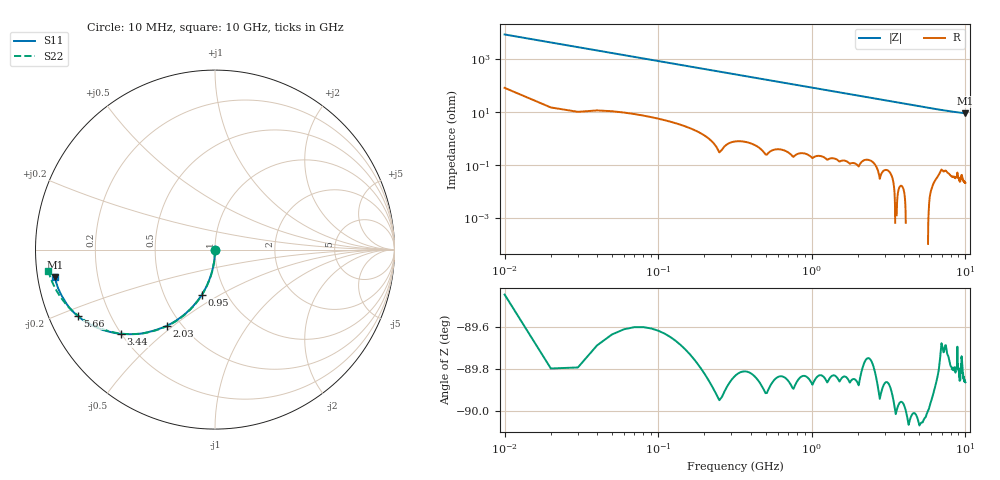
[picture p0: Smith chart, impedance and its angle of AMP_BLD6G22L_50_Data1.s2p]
! Created Fri Sep 09 16:33:03 2011
# ghz S ma R 50
! 2 Port Network Data from SP1.SP block
! freq  magS11  angS11  magS21  angS21  magS12  angS12  magS22  angS22
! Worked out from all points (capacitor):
!   1000 points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, 10 MHz to 10 GHz, reference 50 ohm
!   read as one part in shunt: C = 1.87 pF near 60 MHz
!   lowest |Z| = 9.03 ohm at 10 GHz (marker M1)
!   S11 on the Smith chart (normalised r, x): 10 MHz: 1.00, -0.01; 950 MHz: 0.77, -0.41; 2.03 GHz: 0.42, -0.47; 3.44 GHz: 0.20, -0.37; 5.66 GHz: 0.09, -0.23; 10 GHz: 0.05, -0.08
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0.01  0.002866 -90.6  1 -0.2  1 -0.2  0.00286 -90.7
0.04  0.01146 -91.0  0.9999 -0.7  0.9999 -0.7  0.01144 -91.0
0.07  0.02005 -91.7  0.9997 -1.2  0.9997 -1.2  0.02002 -91.6
0.1  0.02864 -92.2  0.9994 -1.7  0.9994 -1.7  0.02859 -92.1
0.13  0.03722 -92.6  0.9991 -2.2  0.9991 -2.2  0.03716 -92.5
0.16  0.0458 -93.1  0.9987 -2.8  0.9987 -2.8  0.04571 -93.0
0.24  0.06862 -94.3  0.9976 -4.1  0.9976 -4.1  0.06849 -94.2
0.36  0.1026 -96.5  0.9944 -6.2  0.9944 -6.2  0.1024 -96.3
0.52  0.1474 -99.1  0.9888 -8.9  0.9888 -8.9  0.1472 -98.9
0.72  0.202 -102.5  0.9789 -12.3  0.9789 -12.3  0.2019 -102.3
0.95  0.2625 -106.3  0.9642 -16.1  0.9642 -16.1  0.2627 -106.1
1.28  0.3442 -111.6  0.9378 -21.3  0.9378 -21.3  0.3447 -111.3
1.68  0.4336 -117.5  0.8994 -27.3  0.8994 -27.3  0.4346 -117.3
2.03  0.5029 -122.3  0.8623 -32.1  0.8623 -32.1  0.5043 -122.2
2.71  0.6139 -130.6  0.7864 -40.6  0.7864 -40.6  0.6154 -130.7
3.34  0.6922 -137.2  0.7177 -47.3  0.7177 -47.3  0.6936 -137.4
3.44  0.7032 -138.1  0.7074 -48.3  0.7074 -48.3  0.7044 -138.4
5.01  0.8207 -150.2  0.5647 -60.8  0.5647 -60.8  0.8226 -151.0
5.66  0.8489 -154.1  0.5178 -64.7  0.5178 -64.7  0.8533 -155.1
6.67  0.8771 -159.0  0.4578 -69.6  0.4578 -69.6  0.8871 -160.5
8.34  0.898 -165.4  0.3864 -76.2  0.3864 -76.2  0.9194 -167.3
10  0.9048 -170.3  0.3417 -81.4  0.3417 -81.4  0.9361 -172.7
